(* Logix 5000 AddOnInstructionDefinition export CFW900_101151; software revision 20.06 *)

ADD_ON_INSTRUCTION CFW900_101151   (* revision 1.0, ExecutePrescan *)
// 101/151 WEG Advanced Torque
// AOI
// Help:
// Drive setup as follows:
// C9.2.1.1 - 3
// C9.2.1.2 - 7
// C9.2.1.3 - 5
// C9.2.1.4 - 60
// C9.2.1.5 - USER DEFINED
// C9.2.1.6 - USER DEFINED
// C9.2.1.7 - USER DEFINED
// C9.2.2.2 - 100
// C9.2.2.3 - 101
// C9.2.2.4 - 4001
// C9.2.2.5 - 4002
// C9.2.2.6 - USER DEFINED
// C9.2.2.7 - USER DEFINED
// C9.5.1 = 101/151
// C9.5.2 = 1
// C9.5.3 = 7
// C9.5.4 = 1
// C9.5.5 = 7
// C4.1.1 - Ethernet
// C4.1.2 - Inactive
// C4.1.3 - Disable
// C4.2.2.1 - Ethernet
// C4.2.2.2 - Ethernet
// C4.2.2.3 - Ethernet
// C4.2.2.4 - Ethernet
// C4.3.1.2.1 - Keypad
// C4.3.1.2.2 - Ethernet
VAR_INPUT
   ConnectionFaulted : BOOL; {required}   // From CFW900
END_VAR
VAR_IN_OUT
   Inputs : INT[10]; {required}   // Input Assembly From CFW900
   Outputs : INT[10]; {required}   // Output Assembly To CFW900
END_VAR
VAR_INPUT
   cmd_DriveEnable : BOOL; {visible}   // 1 = Enable Operation of Drive 0 = Disable Operation of Drive
   cmd_NetCtrl : BOOL := 1; {visible}   // 1 = Remote (PLC) Control 0 = Local (HMI) Control
   cfg_RampSelect : BOOL; {visible}   // 1 = Ramp 2 (C6.1.4/C61.5) 0 = Ramp 1 (C6.1.1/C6.1.2)
   cmd_Fault_Reset : BOOL; {visible}   // 1 = Fault Reset 0 = No action
   cmd_QuickStop : BOOL := 1; {visible}   // 1 = NO Quick Stop 0 = Quick Stop
   cmd_RunForward : BOOL; {visible}   // 1 = Run Fwd 0 = Stop
   cmd_RunReverse : BOOL; {visible}   // 1 = Run Rev 0 = Stop
   cmd_JogForward : BOOL; {visible}   // 1 = Jog Fwd 0 = No Action / Stop
   cmd_JogReverse : BOOL; {visible}   // 1 = Jog Reverse 0 = No Action / Stop
   set_Speed_Reference : REAL; {required}   // Speed Setpoint (in %)
   set_Torque_Reference : REAL; {required}   // Torque Reference 0-100%
END_VAR
VAR_OUTPUT
   val_RealSpeed : REAL; {access Read Only, visible}   // Current Speed (in %)
   val_RealTorque : REAL; {access Read Only, visible}   // Current Torque
   sts_Connection_Faulted : BOOL; {access Read Only, visible}   // Connection is interrupted status bit
   sts_Faulted : BOOL; {access Read Only, visible}   // 1 = Drive Faulted 0 = Drive not in Fault
   val_FaultCode : DINT; {access Read Only, visible}   // Fault Code 1 from Drive
   sts_Local : BOOL; {access Read Only, visible}   // 1 = Local 0 = Remote
   sts_Connection_Ready : BOOL; {access None, visible}   // Indicates that CFW900 connection is not in a faulted state
   sts_ConfigMode : BOOL; {access Read Only, visible}   // 1 = CFW900 in config mode 0 = CFW900 in operation mode
   sts_Ready : BOOL; {access Read Only, visible}   // 1 = Drive is ready to operate (states Ready, Enabled or Stopping) 0 = Drive is not ready to operate
   sts_STO : BOOL; {access Read Only, visible}   // 1 = Safe Torque Off (STO) Active 0 = STO Not Active
   sts_NoQuickStop : BOOL; {access Read Only, visible}   // 1 = No quick stop commanded 0 = Quick Stop commanded
   sts_Ctrl_from_net : BOOL; {access Read Only, visible}   // 1 = drive is controlled remotely (PLC) 0 = drive is controlled locally (HMI)
   sts_Ramp2_Selected : BOOL; {access None, visible}   // 1 = Ramp 2 rates selected 0 = Ramp 1 rates selected
   sts_RunCommand : BOOL; {access Read Only, visible}   // 1 = Commanded to run 0 = Not commanded to run
   sts_RunningForward : BOOL; {access Read Only, visible}   // 1 = CFW900 Running Forward 0 = CFW900 Stopped
   sts_RunningReverse : BOOL; {access Read Only, visible}   // 1 = CFW900 Running Reverse 0 = CFW900 not running reverse
   sts_STO_Fault : BOOL; {access Read Only, visible}   // STO has been tripped while run cmd active
   val_OutputCurrent : REAL; {access Read Only, visible}   // Output current from Drive to Motor
   val_OutputFreq : REAL; {access Read Only, visible}   // Output Frequency in Hz
   val_OutputVoltage : DINT; {access Read Only, visible}   // Voltage Applied to Motor
END_VAR
VAR_INPUT
   set_Accel : REAL := 10.0; {required}   // Acceleration Ramp time (in seconds)
   set_Decel : REAL := 10.0; {required}   // Deceleration Ramp setpoint (0.1-999.9) in seconds
   set_IncRamp : REAL := 10.0; {access None, required}   // Torque Control Ramp 0.1 to 999.9s
   set_DecRamp : REAL := 10.0; {required}   // Torque Control Ramp 0.1 to 999.9s
END_VAR
VAR
   FailToStart : TIMER; {access None}
   Wrk_Run1 : BOOL; {access None}   // Internal bit to signal run1
   Wrk_Run2 : BOOL; {access None}   // Internal bit to signal run2
   FailToStop : TIMER; {access None}
   Wrk_Jog2 : BOOL; {access None}   // Internal bit for reverse Jog
   Wrk_Jog1 : BOOL; {access None}   // Internal Bit for forward Jog
   TempReal : REAL; {access None}
   TempDINT : DINT; {access None}
END_VAR

ROUTINE Logic   (* ladder *)
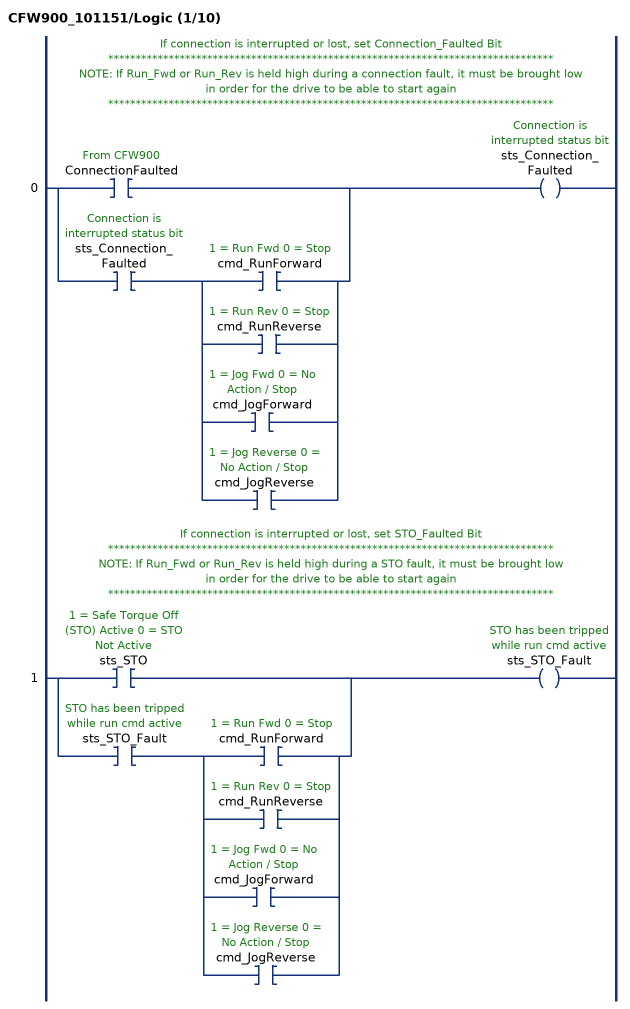
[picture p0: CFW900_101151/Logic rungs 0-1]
   // If connection is interrupted or lost, set Connection_Faulted Bit
   // *********************************************************************************
   // NOTE: If Run_Fwd or Run_Rev is held high during a connection fault, it must be brought low
   // in order for the drive to be able to start again
   // *********************************************************************************
   0: [XIC(ConnectionFaulted) ,XIC(sts_Connection_Faulted) [XIC(cmd_RunForward) ,XIC(cmd_RunReverse) ,XIC(cmd_JogForward) ,XIC(cmd_JogReverse) ] ]OTE(sts_Connection_Faulted);
   // If connection is interrupted or lost, set STO_Faulted Bit
   // *********************************************************************************
   // NOTE: If Run_Fwd or Run_Rev is held high during a STO fault, it must be brought low
   // in order for the drive to be able to start again
   // *********************************************************************************
   1: [XIC(sts_STO) ,XIC(sts_STO_Fault) [XIC(cmd_RunForward) ,XIC(cmd_RunReverse) ,XIC(cmd_JogForward) ,XIC(cmd_JogReverse) ] ]OTE(sts_STO_Fault);
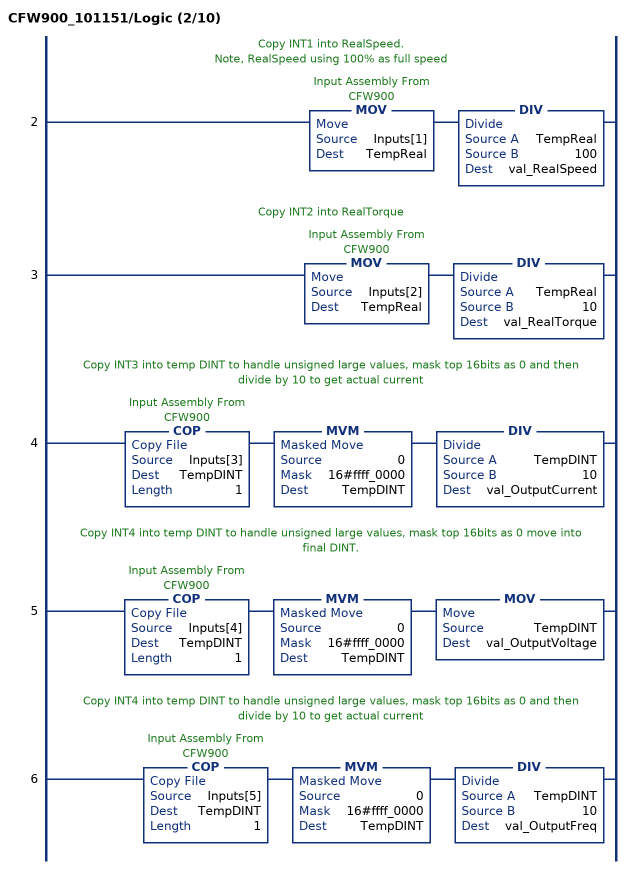
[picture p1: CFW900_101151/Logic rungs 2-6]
   // Copy INT1 into RealSpeed.
   // Note, RealSpeed using 100% as full speed
   2: MOV(Inputs[1],TempReal)DIV(TempReal,100,val_RealSpeed);
   // Copy INT2 into RealTorque
   3: MOV(Inputs[2],TempReal)DIV(TempReal,10,val_RealTorque);
   // Copy INT3 into temp DINT to handle unsigned large values, mask top 16bits as 0 and then divide by 10 to get actual current
   4: COP(Inputs[3],TempDINT,1)MVM(0,16#ffff_0000,TempDINT)DIV(TempDINT,10,val_OutputCurrent);
   // Copy INT4 into temp DINT to handle unsigned large values, mask top 16bits as 0 move into final DINT.
   5: COP(Inputs[4],TempDINT,1)MVM(0,16#ffff_0000,TempDINT)MOV(TempDINT,val_OutputVoltage);
   // Copy INT4 into temp DINT to handle unsigned large values, mask top 16bits as 0 and then divide by 10 to get actual current
   6: COP(Inputs[5],TempDINT,1)MVM(0,16#ffff_0000,TempDINT)DIV(TempDINT,10,val_OutputFreq);
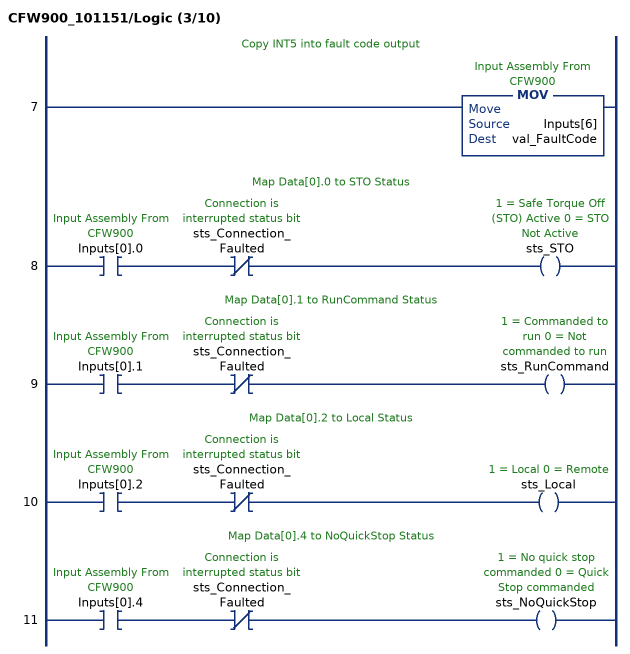
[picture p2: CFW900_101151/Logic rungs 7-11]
   // Copy INT5 into fault code output
   7: MOV(Inputs[6],val_FaultCode);
   // Map Data[0].0 to STO Status
   8: XIC(Inputs[0].0)XIO(sts_Connection_Faulted)OTE(sts_STO);
   // Map Data[0].1 to RunCommand Status
   9: XIC(Inputs[0].1)XIO(sts_Connection_Faulted)OTE(sts_RunCommand);
   // Map Data[0].2 to Local Status
   10: XIC(Inputs[0].2)XIO(sts_Connection_Faulted)OTE(sts_Local);
   // Map Data[0].4 to NoQuickStop Status
   11: XIC(Inputs[0].4)XIO(sts_Connection_Faulted)OTE(sts_NoQuickStop);
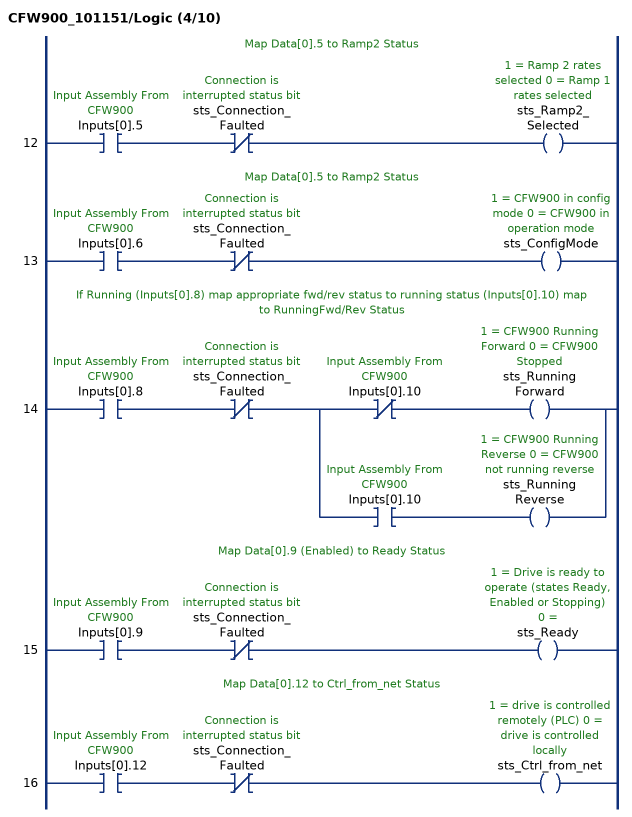
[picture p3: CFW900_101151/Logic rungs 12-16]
   // Map Data[0].5 to Ramp2 Status
   12: XIC(Inputs[0].5)XIO(sts_Connection_Faulted)OTE(sts_Ramp2_Selected);
   // Map Data[0].5 to Ramp2 Status
   13: XIC(Inputs[0].6)XIO(sts_Connection_Faulted)OTE(sts_ConfigMode);
   // If Running (Inputs[0].8) map appropriate fwd/rev status to running status (Inputs[0].10) map to RunningFwd/Rev Status
   14: XIC(Inputs[0].8)XIO(sts_Connection_Faulted)[XIO(Inputs[0].10) OTE(sts_RunningForward) ,XIC(Inputs[0].10) OTE(sts_RunningReverse) ];
   // Map Data[0].9 (Enabled) to Ready Status
   15: XIC(Inputs[0].9)XIO(sts_Connection_Faulted)OTE(sts_Ready);
   // Map Data[0].12 to Ctrl_from_net Status
   16: XIC(Inputs[0].12)XIO(sts_Connection_Faulted)OTE(sts_Ctrl_from_net);
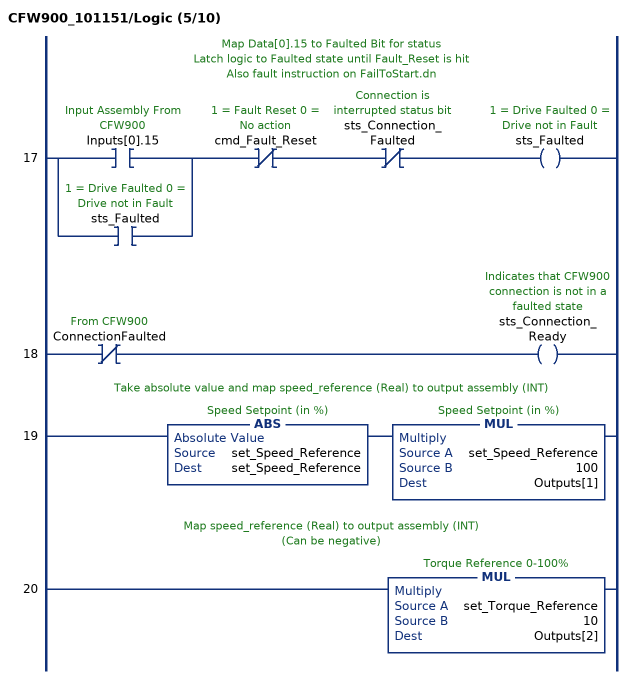
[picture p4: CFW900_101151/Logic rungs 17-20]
   // Map Data[0].15 to Faulted Bit for status
   // Latch logic to Faulted state until Fault_Reset is hit
   // Also fault instruction on FailToStart.dn
   17: [XIC(Inputs[0].15) ,XIC(sts_Faulted) ]XIO(cmd_Fault_Reset)XIO(sts_Connection_Faulted)OTE(sts_Faulted);
   18: XIO(ConnectionFaulted)OTE(sts_Connection_Ready);
   // Take absolute value and map speed_reference (Real) to output assembly (INT)
   19: ABS(set_Speed_Reference,set_Speed_Reference)MUL(set_Speed_Reference,100,Outputs[1]);
   // Map speed_reference (Real) to output assembly (INT)
   // (Can be negative)
   20: MUL(set_Torque_Reference,10,Outputs[2]);
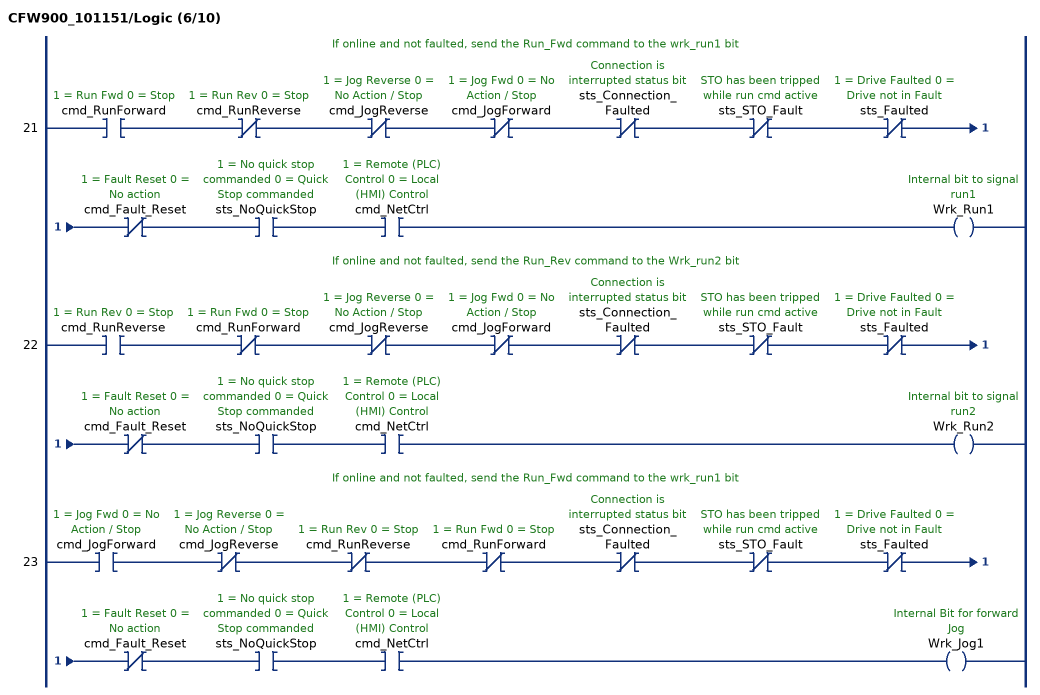
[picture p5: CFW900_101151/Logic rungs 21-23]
   // If online and not faulted, send the Run_Fwd command to the wrk_run1 bit
   21: XIC(cmd_RunForward)XIO(cmd_RunReverse)XIO(cmd_JogReverse)XIO(cmd_JogForward)XIO(sts_Connection_Faulted)XIO(sts_STO_Fault)XIO(sts_Faulted)XIO(cmd_Fault_Reset)XIC(sts_NoQuickStop)XIC(cmd_NetCtrl)OTE(Wrk_Run1);
   // If online and not faulted, send the Run_Rev command to the Wrk_run2 bit
   22: XIC(cmd_RunReverse)XIO(cmd_RunForward)XIO(cmd_JogReverse)XIO(cmd_JogForward)XIO(sts_Connection_Faulted)XIO(sts_STO_Fault)XIO(sts_Faulted)XIO(cmd_Fault_Reset)XIC(sts_NoQuickStop)XIC(cmd_NetCtrl)OTE(Wrk_Run2);
   // If online and not faulted, send the Run_Fwd command to the wrk_run1 bit
   23: XIC(cmd_JogForward)XIO(cmd_JogReverse)XIO(cmd_RunReverse)XIO(cmd_RunForward)XIO(sts_Connection_Faulted)XIO(sts_STO_Fault)XIO(sts_Faulted)XIO(cmd_Fault_Reset)XIC(sts_NoQuickStop)XIC(cmd_NetCtrl)OTE(Wrk_Jog1);
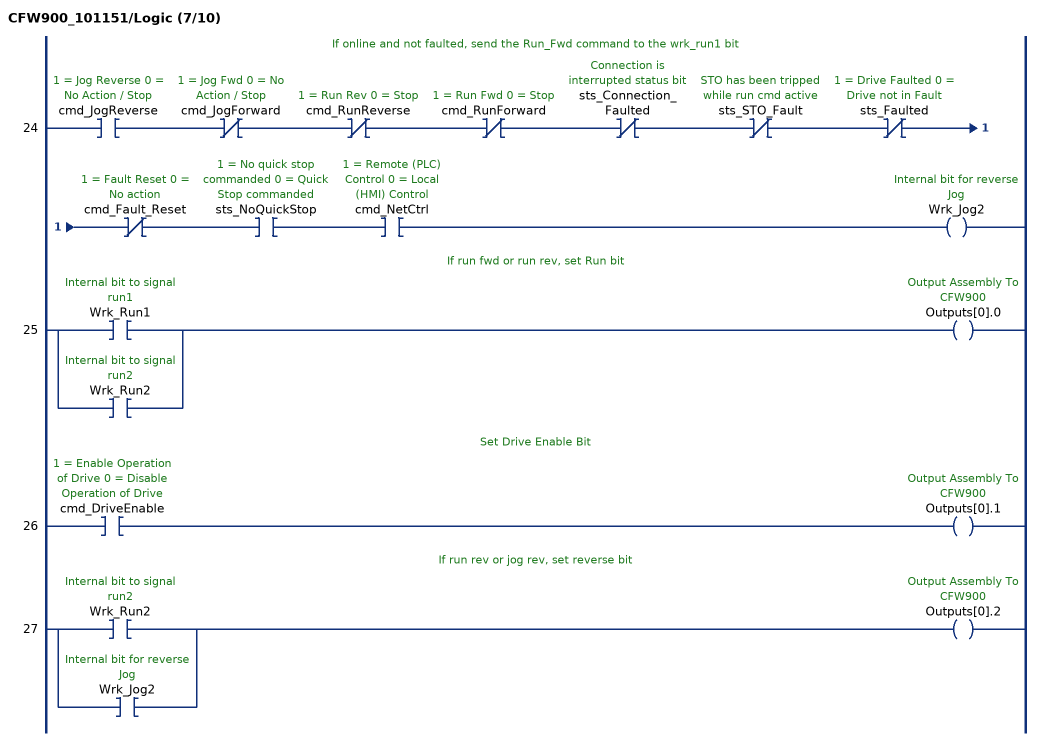
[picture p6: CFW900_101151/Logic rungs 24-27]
   // If online and not faulted, send the Run_Fwd command to the wrk_run1 bit
   24: XIC(cmd_JogReverse)XIO(cmd_JogForward)XIO(cmd_RunReverse)XIO(cmd_RunForward)XIO(sts_Connection_Faulted)XIO(sts_STO_Fault)XIO(sts_Faulted)XIO(cmd_Fault_Reset)XIC(sts_NoQuickStop)XIC(cmd_NetCtrl)OTE(Wrk_Jog2);
   // If run fwd or run rev, set Run bit
   25: [XIC(Wrk_Run1) ,XIC(Wrk_Run2) ]OTE(Outputs[0].0);
   // Set Drive Enable Bit
   26: XIC(cmd_DriveEnable)OTE(Outputs[0].1);
   // If run rev or jog rev, set reverse bit
   27: [XIC(Wrk_Run2) ,XIC(Wrk_Jog2) ]OTE(Outputs[0].2);
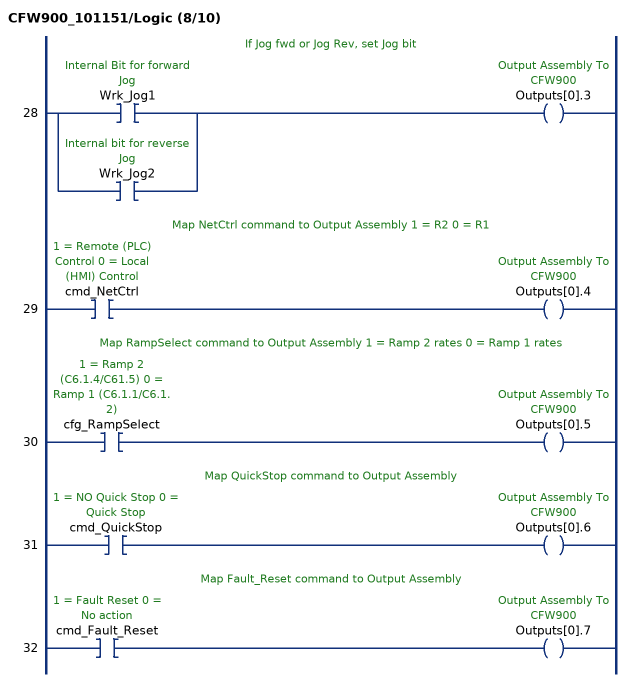
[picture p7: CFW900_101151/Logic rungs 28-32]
   // If Jog fwd or Jog Rev, set Jog bit
   28: [XIC(Wrk_Jog1) ,XIC(Wrk_Jog2) ]OTE(Outputs[0].3);
   // Map NetCtrl command to Output Assembly 1 = R2 0 = R1
   29: XIC(cmd_NetCtrl)OTE(Outputs[0].4);
   // Map RampSelect command to Output Assembly 1 = Ramp 2 rates 0 = Ramp 1 rates
   30: XIC(cfg_RampSelect)OTE(Outputs[0].5);
   // Map QuickStop command to Output Assembly
   31: XIC(cmd_QuickStop)OTE(Outputs[0].6);
   // Map Fault_Reset command to Output Assembly
   32: XIC(cmd_Fault_Reset)OTE(Outputs[0].7);
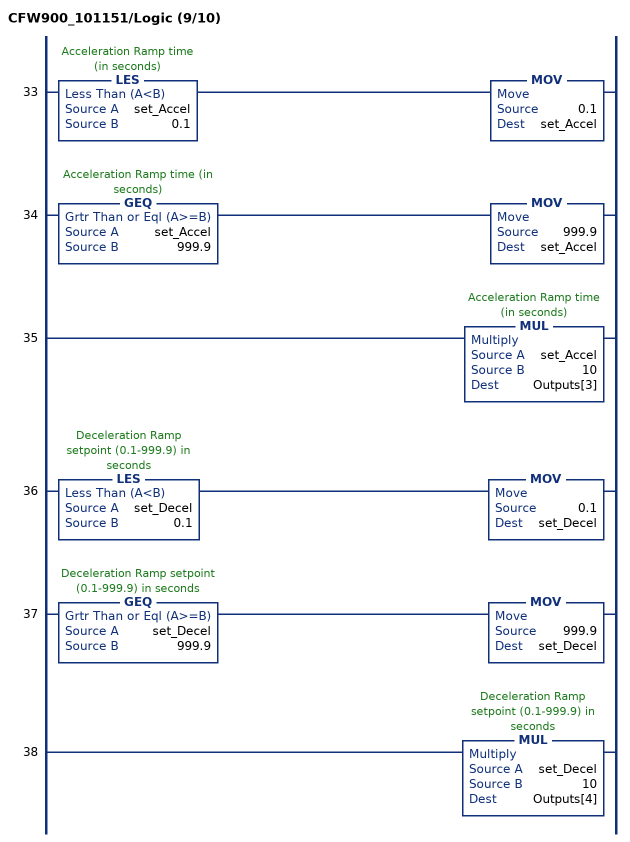
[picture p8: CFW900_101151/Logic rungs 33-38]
   33: LES(set_Accel,0.1)MOV(0.1,set_Accel);
   34: GEQ(set_Accel,999.9)MOV(999.9,set_Accel);
   35: MUL(set_Accel,10,Outputs[3]);
   36: LES(set_Decel,0.1)MOV(0.1,set_Decel);
   37: GEQ(set_Decel,999.9)MOV(999.9,set_Decel);
   38: MUL(set_Decel,10,Outputs[4]);
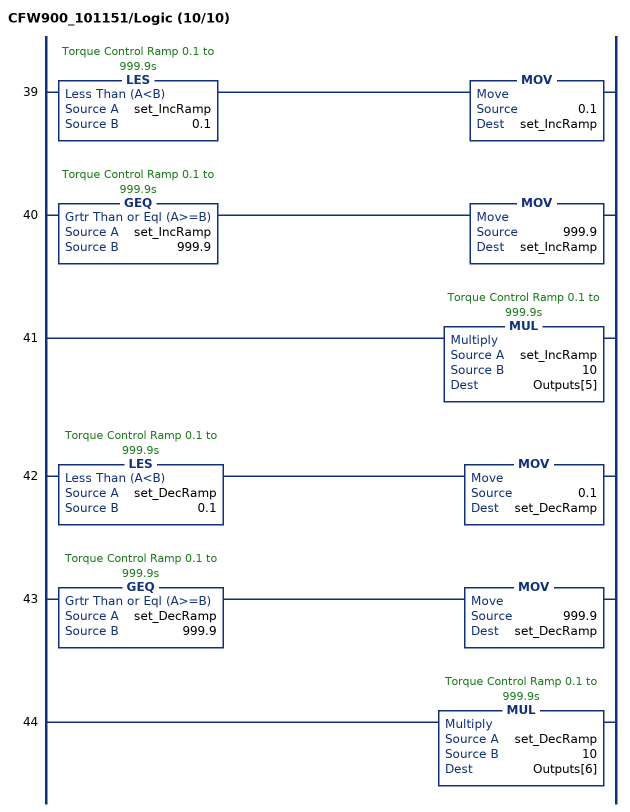
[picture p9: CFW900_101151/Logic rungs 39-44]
   39: LES(set_IncRamp,0.1)MOV(0.1,set_IncRamp);
   40: GEQ(set_IncRamp,999.9)MOV(999.9,set_IncRamp);
   41: MUL(set_IncRamp,10,Outputs[5]);
   42: LES(set_DecRamp,0.1)MOV(0.1,set_DecRamp);
   43: GEQ(set_DecRamp,999.9)MOV(999.9,set_DecRamp);
   44: MUL(set_DecRamp,10,Outputs[6]);
END_ROUTINE

ROUTINE Prescan   (* ladder *)
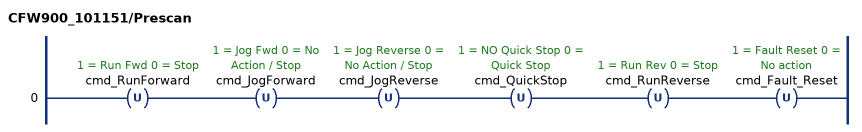
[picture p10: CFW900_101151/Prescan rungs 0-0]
   0: OTU(cmd_RunForward)OTU(cmd_JogForward)OTU(cmd_JogReverse)OTU(cmd_QuickStop)OTU(cmd_RunReverse)OTU(cmd_Fault_Reset);
END_ROUTINE
END_ADD_ON_INSTRUCTION
